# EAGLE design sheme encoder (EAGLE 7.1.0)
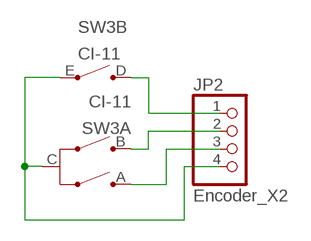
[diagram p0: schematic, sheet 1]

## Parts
JP2  Encoder_X2  PINHD-1X4  [1X04]
SW3  CI-11  [CI-11]

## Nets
N$3: JP2.1 SW3.D(B:D)
N$4: JP2.2 SW3.B(A:B)
N$5: JP2.3 SW3.A(A:A)
N$6: JP2.4 SW3.C(A:C) SW3.E(B:E)

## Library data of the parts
JP2 = pinhead:PINHD-1X4: PIN HEADER
SW3 = piher:CI-11: 11mm Incemental Encoder Source: www.piher.net .. 04-CI-11v04.pdf; OC_FARNELL: unknown; OC_NEWARK: unknown

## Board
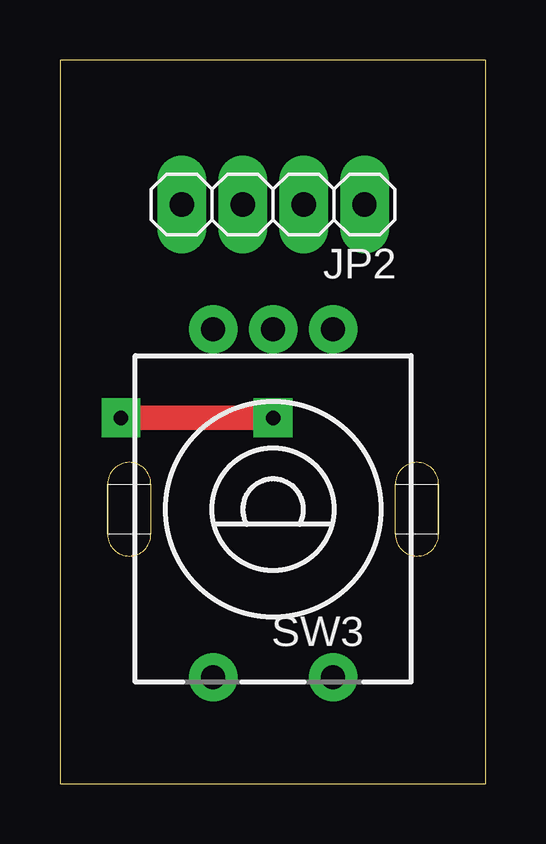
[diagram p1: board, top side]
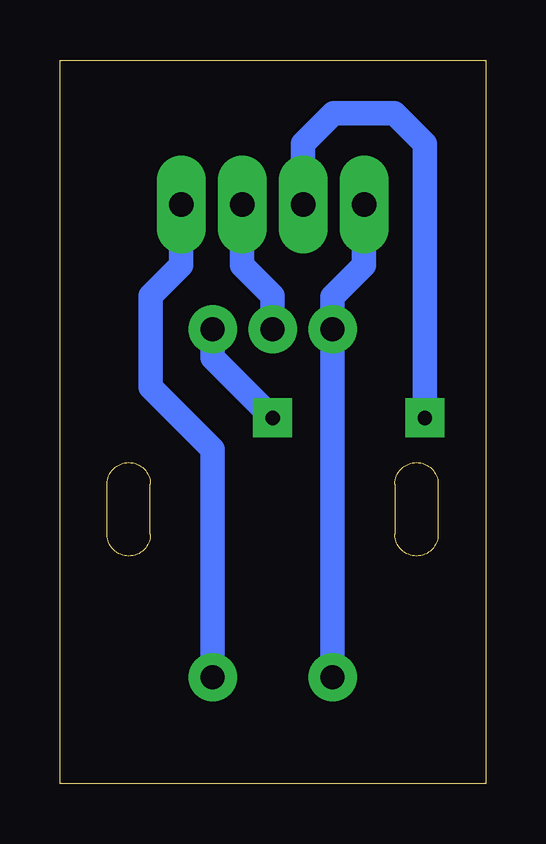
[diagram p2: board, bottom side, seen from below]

Size 17.76 x 30.15 mm. Coordinates in mm from the lower left corner, seen from the top.
Outline: 0,0 17.76,0 17.76,30.15 0,30.15 0,0
Copper layers (1*16): Top 0.035mm / dielectric 1.5mm / Bottom 0.035mm
Design rules "default *": minimum track width 12mil, minimum drill 20mil, track to track 12mil, track to pad 12mil, pad to pad 12mil, via to via 12mil, smd to smd 8mil, copper to edge 40mil, drill to drill 20mil, minimum pad ring 20mil, minimum via ring 20mil, stop-mask expansion 4mil, vias tented up to drill 0mil, thermal gap 10mil

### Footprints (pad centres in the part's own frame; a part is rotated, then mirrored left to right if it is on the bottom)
1X04 = drill 1.016 long: 1 -3.81,0; 2 -1.27,0; 3 1.27,0; 4 3.81,0
CI-11 = drill 1 pad 1.676: A -2.5,-7.5; B 0,-7.5; C 2.5,-7.5; D -2.5,7; E 2.5,7

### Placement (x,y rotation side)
JP2  8.89,24.13 180 top
SW3  8.89,11.43 180 top

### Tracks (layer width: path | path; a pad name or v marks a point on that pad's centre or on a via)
N$3
  Bottom 1.016: SW3.D 11.39,13.93 13.97,16.51 13.97,20.32 12.7,21.59 JP2.1
N$4
  Bottom 1.016: SW3.B 8.89,20.32 10.16,21.59 JP2.2
N$5  (via drill 0.6)
  Top 1.016: v8.89,15.24 v2.54,15.24
  Bottom 1.016: SW3.A 11.39,17.74 v8.89,15.24 | v2.54,15.24 2.54,26.67 3.81,27.94 6.35,27.94 7.62,26.67 JP2.3
N$6
  Bottom 1.016: SW3.E SW3.C 6.39,20.28 5.08,21.59 JP2.4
